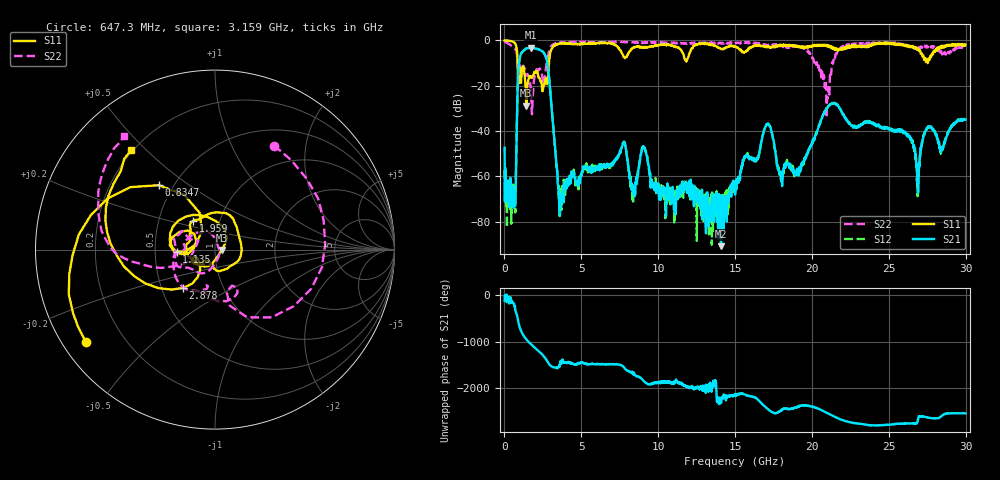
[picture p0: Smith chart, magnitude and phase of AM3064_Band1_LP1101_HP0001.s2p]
# Hz S DB R 50.0
!freq dBS11 angS11 dBS21 angS21 dBS12 angS12 dBS22 angS22
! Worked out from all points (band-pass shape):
!   1600 points, 10 MHz to 29.98 GHz, reference 50 ohm
!   highest |S21| = -3.25 dB at 1.716 GHz (marker M1); lowest = -90.9 dB at 14.09 GHz (marker M2)
!   |S21| within 3 dB of the highest: 1.056 GHz to 2.625 GHz (1.569 GHz wide, 85.2 % of centre)
!   lowest |S11| = -28.8 dB at 1.416 GHz (marker M3), VSWR 1.08, Z = 53.8 - j0.195 ohm
!   |S11| at or under -10 dB: 857.6 MHz to 2.892 GHz (2.035 GHz wide, 109 % of centre); 27.5253 GHz to 27.52778 GHz (2.482 MHz wide, 0.00902 % of centre)
!   |S22| runs from -34.2 to -0.4 dB; largest |S21 - S12| = 0.0093
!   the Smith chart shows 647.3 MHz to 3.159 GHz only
!   S11 on the Smith chart (normalised r, x): 647.3 MHz: 0.07, -0.32; 834.7 MHz: 0.42, +0.39; 1.135 GHz: 0.65, -0.02; 1.959 GHz: 0.75, +0.25; 2.878 GHz: 0.64, -0.30; 3.159 GHz: 0.19, +0.45
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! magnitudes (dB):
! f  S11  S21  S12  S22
! 10 MHz  -0.1  -47.4  -57.1  -0.4
! 647.3 MHz  -1.1  -68.0  -66.5  -3.5
! 834.7 MHz  -6.4  -27.6  -27.5  -7.6
! 1.135 GHz  -13.4  -5.3  -5.2  -12.6
! 1.416 GHz  -28.8  -3.6  -3.6  -15.3
! 1.716 GHz  -15.9  -3.2  -3.2  -21.9
! 1.959 GHz  -13.9  -3.5  -3.5  -16.3
! 2.878 GHz  -11.1  -14.6  -14.6  -5.2
! 3.159 GHz  -2.8  -36.9  -37.0  -1.8
! 3.628 GHz  -1.4  -71.7  -71.1  -1.1
! 5.015 GHz  -1.5  -59.6  -59.8  -0.7
! 9.063 GHz  -3.0  -46.9  -47.1  -1.1
! 10 GHz  -2.1  -63.2  -63.5  -1.0
! 14.09 GHz  -3.8  -90.9  -70.1  -1.3
! 15 GHz  -2.8  -68.1  -64.4  -1.3
! 17.09 GHz  -2.7  -37.0  -37.1  -2.0
! 17.95 GHz  -2.3  -59.1  -59.4  -2.1
! 19.99 GHz  -2.8  -45.9  -45.7  -7.0
! 20.98 GHz  -2.1  -29.9  -29.8  -26.3
! 25 GHz  -1.1  -39.3  -38.9  -1.2
! 26.87 GHz  -4.1  -64.0  -68.8  -3.0
! 29.98 GHz  -1.9  -35.0  -34.8  -2.8
